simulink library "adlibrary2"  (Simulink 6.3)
undefined symbols (not defined in the file or in its folder): adlibrary2, ADM, DDRII, II, no_bitstream, SRAM, XP, XRC
libraries: xbsIndex_r4 x297, adlibrary2_d2sram_0 x5, adlibrary2 x5, adlibrary2_ddr_xpi0 x4, adlibrary2_ddr_xpl x3, adlibrary2_xpl32 x1, adlibrary2_xpl64 x1, adlibrary2_zbt64 x1, adlibrary2_zbt4_0 x1, adlibrary2_zbt4_1 x1, adlibrary2_zbt4_2 x1, adlibrary2_zbt4_3 x1
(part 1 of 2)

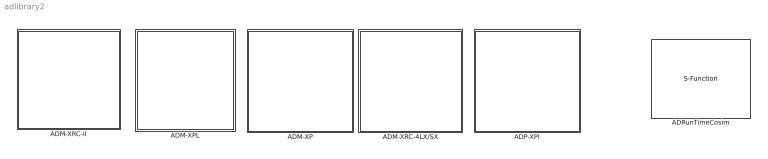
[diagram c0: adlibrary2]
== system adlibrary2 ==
  ADM-XP : Subsystem
  ADM-XPL : Subsystem
  ADM-XRC-4LX/SX : Subsystem  AncestorBlock=adlibrary2/ADM-XRC-II
  ADM-XRC-II : Subsystem
  ADP-XPI : Subsystem
  ADRunTimeCosim : S-Function  FunctionName=adcosim  Parameters='',index,bitstream,freq,single_step,shared  mask{index=0, bitstream=no_bitstream, freq=50, single_step=off, shared=None}
      mask prompts: index "Card Index"; freq "Clock Frequency"; single_step "Single Step"; shared "Share Access"

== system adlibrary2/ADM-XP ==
  DDR SDRAM 0 : Subsystem  mask{memsize=1}
      mask prompts: memsize "Simulation RAM Size (Mb)"
  DDR SDRAM 1 : Subsystem  mask{memsize=1}
      mask prompts: memsize "Simulation RAM Size (Mb)"
  DDRII SRAM 0 : Subsystem
  DDRII SRAM 1 : Subsystem  AncestorBlock=adlibrary2/ADM-XP/DDRII SRAM 0
  DDRII SRAM 2 : Subsystem
  DDRII SRAM 3 : Subsystem
  XPL 32 Bit Interface : adlibrary2/ADM-XPL/XPL 32 Bit Interface  program='load myprogram.txt'  clock_ratio=1.5
  XPL 64 Bit Interface : adlibrary2/ADM-XPL/XPL 64 Bit Interface  program='load myprogram.txt'  clock_ratio=1.5

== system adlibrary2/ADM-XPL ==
  DDR SDRAM : Subsystem  mask{memsize=1}
      mask prompts: memsize "Simulation RAM Size (Mb)"
  XPL 32 Bit Interface : Subsystem  mask{program='load myprogram.txt', clock_ratio=1.5}
      mask prompts: program "Local Bus Script Program"; clock_ratio "Clock Ratio"
  XPL 64 Bit Interface : Subsystem  mask{program='load myprogram.txt', clock_ratio=1.5}
      mask prompts: program "Local Bus Script Program"; clock_ratio "Clock Ratio"
  ZBT SRAM 64 : Subsystem

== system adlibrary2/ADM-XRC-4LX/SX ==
  PLX 32 Bit Interface : adlibrary2/ADM-XRC-II/PLX 32 Bit Interface  program='load myprogram.txt'  clock_ratio=1.5
  ZBT SRAM 0 : Subsystem
  ZBT SRAM 1 : Subsystem
  ZBT SRAM 2 : Subsystem
  ZBT SRAM 3 : Subsystem
  ZBT SRAM 4 : Subsystem
  ZBT SRAM 5 : Subsystem

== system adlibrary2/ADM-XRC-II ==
  PLX 32 Bit Interface : Subsystem  mask{program='load myprogram.txt', clock_ratio=1.5}
      mask prompts: program "Local Bus Script Program"; clock_ratio "Clock Ratio"
  "XRM DDR SDRAM " : Subsystem  mask{memsize=1}
      mask prompts: memsize "Simulation RAM Size (Mb)"
  ZBT SRAM 0 : Subsystem
  ZBT SRAM 1 : Subsystem
  ZBT SRAM 2 : Subsystem
  ZBT SRAM 3 : Subsystem
  ZBT SRAM 4 : Subsystem
  ZBT SRAM 5 : Subsystem

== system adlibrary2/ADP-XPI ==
  DDR SDRAM 0 : Subsystem  mask{memsize=1}
      mask prompts: memsize "Simulation RAM Size (Mb)"
  DDR SDRAM 1 : Subsystem  mask{memsize=1}
      mask prompts: memsize "Simulation RAM Size (Mb)"
  DDR SDRAM 2 : Subsystem  mask{memsize=1}
      mask prompts: memsize "Simulation RAM Size (Mb)"
  DDR SDRAM 3 : Subsystem  mask{memsize=1}
      mask prompts: memsize "Simulation RAM Size (Mb)"
  DDRII SRAM 0 : Subsystem
  XPL 32 Bit Interface : adlibrary2/ADM-XPL/XPL 32 Bit Interface  program='load myprogram.txt'  clock_ratio=1.5
  XPL 64 Bit Interface : adlibrary2/ADM-XPL/XPL 64 Bit Interface  program='load myprogram.txt'  clock_ratio=1.5

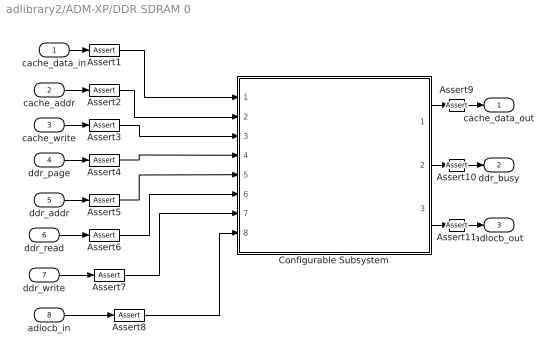
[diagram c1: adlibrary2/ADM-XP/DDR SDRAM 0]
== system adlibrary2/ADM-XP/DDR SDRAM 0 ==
  cache_data_in : Inport
  cache_addr : Inport  Port=2
  cache_write : Inport  Port=3
  ddr_page : Inport  Port=4
  ddr_addr : Inport  Port=5
  ddr_read : Inport  Port=6
  ddr_write : Inport  Port=7
  adlocb_in : Inport  Port=8
  Assert{1..11} (11 alike) : xbsIndex_r4/Assert  assert_type=off  type_source=Explicitly  arith_type="Signed  (2's comp)"  n_bits=16  bin_pt=14  assert_rate=on  rate_source=Explicitly  period=1  output_port=on  block_type=assert
  Configurable Subsystem : Subsystem  Tag=configX  BlockChoice=DDR SDRAM 32bit Simulation  mask{memsize=memsize}
      mask prompts: memsize "Simulation Ram Size (Mb)"
  cache_data_out : Outport
  ddr_busy : Outport  Port=2
  adlocb_out : Outport  Port=3
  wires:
  Configurable Subsystem/3(adlocb_out) -> Assert11/1
  Configurable Subsystem/2(ddr_busy) -> Assert10/1
  Configurable Subsystem/1(cache_data_out) -> Assert9/1
  cache_data_in/1 -> Assert1/1
  cache_addr/1 -> Assert2/1
  cache_write/1 -> Assert3/1
  ddr_page/1 -> Assert4/1
  ddr_addr/1 -> Assert5/1
  ddr_read/1 -> Assert6/1
  ddr_write/1 -> Assert7/1
  adlocb_in/1 -> Assert8/1
  Assert1/1 -> Configurable Subsystem/1(cache_data_in)
  Assert2/1 -> Configurable Subsystem/2(cache_addr)
  Assert3/1 -> Configurable Subsystem/3(cache_write)
  Assert4/1 -> Configurable Subsystem/4(ddr_page)
  Assert5/1 -> Configurable Subsystem/5(ddr_addr)
  Assert6/1 -> Configurable Subsystem/6(ddr_read)
  Assert7/1 -> Configurable Subsystem/7(ddr_write)
  Assert8/1 -> Configurable Subsystem/8(adlocb_in)
  Assert9/1 -> cache_data_out/1
  Assert10/1 -> ddr_busy/1
  Assert11/1 -> adlocb_out/1

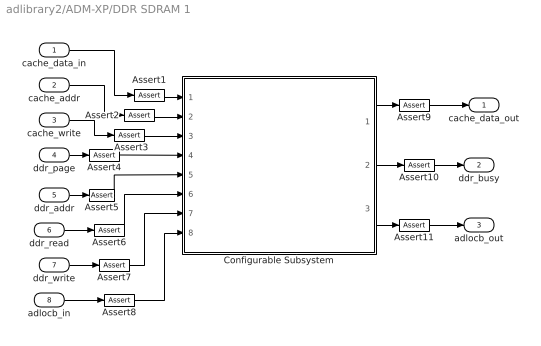
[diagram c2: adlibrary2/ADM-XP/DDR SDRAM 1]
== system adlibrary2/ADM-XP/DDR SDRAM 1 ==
  cache_data_in : Inport
  cache_addr : Inport  Port=2
  cache_write : Inport  Port=3
  ddr_page : Inport  Port=4
  ddr_addr : Inport  Port=5
  ddr_read : Inport  Port=6
  ddr_write : Inport  Port=7
  adlocb_in : Inport  Port=8
  Assert{1..11} (11 alike) : xbsIndex_r4/Assert  assert_type=off  type_source=Explicitly  arith_type="Signed  (2's comp)"  n_bits=16  bin_pt=14  assert_rate=on  rate_source=Explicitly  period=1  output_port=on  block_type=assert
  Configurable Subsystem : Subsystem  Tag=configX  BlockChoice=DDR SDRAM 32bit Simulation  mask{memsize=memsize}
      mask prompts: memsize "Simulation Ram Size (Mb)"
  cache_data_out : Outport
  ddr_busy : Outport  Port=2
  adlocb_out : Outport  Port=3
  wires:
  Configurable Subsystem/3(adlocb_out) -> Assert11/1
  Configurable Subsystem/2(ddr_busy) -> Assert10/1
  Configurable Subsystem/1(cache_data_out) -> Assert9/1
  cache_data_in/1 -> Assert1/1
  cache_addr/1 -> Assert2/1
  cache_write/1 -> Assert3/1
  ddr_page/1 -> Assert4/1
  ddr_addr/1 -> Assert5/1
  ddr_read/1 -> Assert6/1
  ddr_write/1 -> Assert7/1
  adlocb_in/1 -> Assert8/1
  Assert1/1 -> Configurable Subsystem/1(cache_data_in)
  Assert2/1 -> Configurable Subsystem/2(cache_addr)
  Assert3/1 -> Configurable Subsystem/3(cache_write)
  Assert4/1 -> Configurable Subsystem/4(ddr_page)
  Assert5/1 -> Configurable Subsystem/5(ddr_addr)
  Assert6/1 -> Configurable Subsystem/6(ddr_read)
  Assert7/1 -> Configurable Subsystem/7(ddr_write)
  Assert8/1 -> Configurable Subsystem/8(adlocb_in)
  Assert9/1 -> cache_data_out/1
  Assert10/1 -> ddr_busy/1
  Assert11/1 -> adlocb_out/1

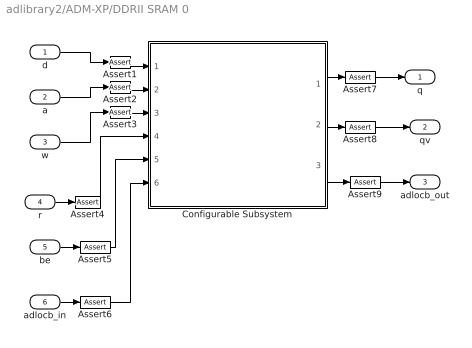
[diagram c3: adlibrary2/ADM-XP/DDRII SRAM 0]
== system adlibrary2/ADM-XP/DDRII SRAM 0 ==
  d : Inport
  a : Inport  Port=2
  w : Inport  Port=3
  r : Inport  Port=4
  be : Inport  Port=5
  adlocb_in : Inport  Port=6
  Assert{1..9} (9 alike) : xbsIndex_r4/Assert  assert_type=off  type_source=Explicitly  arith_type="Signed  (2's comp)"  n_bits=16  bin_pt=14  assert_rate=on  rate_source=Explicitly  period=1  output_port=on  block_type=assert
  Configurable Subsystem : Subsystem  Tag=configX  BlockChoice=DDRII SRAM Simulation
  q : Outport
  qv : Outport  Port=2
  adlocb_out : Outport  Port=3
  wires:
  Configurable Subsystem/1(q) -> Assert7/1
  d/1 -> Assert1/1
  a/1 -> Assert2/1
  w/1 -> Assert3/1
  r/1 -> Assert4/1
  be/1 -> Assert5/1
  adlocb_in/1 -> Assert6/1
  Configurable Subsystem/3(adlocb_out) -> Assert9/1
  Configurable Subsystem/2(qv) -> Assert8/1
  Assert1/1 -> Configurable Subsystem/1(d)
  Assert2/1 -> Configurable Subsystem/2(a)
  Assert3/1 -> Configurable Subsystem/3(w)
  Assert4/1 -> Configurable Subsystem/4(r)
  Assert5/1 -> Configurable Subsystem/5(be)
  Assert6/1 -> Configurable Subsystem/6(adlocb_in)
  Assert7/1 -> q/1
  Assert8/1 -> qv/1
  Assert9/1 -> adlocb_out/1

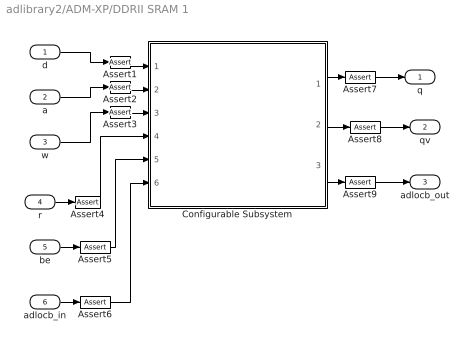
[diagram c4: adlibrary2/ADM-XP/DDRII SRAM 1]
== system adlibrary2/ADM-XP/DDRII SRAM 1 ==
  d : Inport
  a : Inport  Port=2
  w : Inport  Port=3
  r : Inport  Port=4
  be : Inport  Port=5
  adlocb_in : Inport  Port=6
  Assert{1..9} (9 alike) : xbsIndex_r4/Assert  assert_type=off  type_source=Explicitly  arith_type="Signed  (2's comp)"  n_bits=16  bin_pt=14  assert_rate=on  rate_source=Explicitly  period=1  output_port=on  block_type=assert
  Configurable Subsystem : Subsystem  Tag=configX  BlockChoice=DDRII SRAM Simulation
  q : Outport
  qv : Outport  Port=2
  adlocb_out : Outport  Port=3
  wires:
  Configurable Subsystem/1(q) -> Assert7/1
  d/1 -> Assert1/1
  a/1 -> Assert2/1
  w/1 -> Assert3/1
  r/1 -> Assert4/1
  be/1 -> Assert5/1
  adlocb_in/1 -> Assert6/1
  Configurable Subsystem/3(adlocb_out) -> Assert9/1
  Configurable Subsystem/2(qv) -> Assert8/1
  Assert1/1 -> Configurable Subsystem/1(d)
  Assert2/1 -> Configurable Subsystem/2(a)
  Assert3/1 -> Configurable Subsystem/3(w)
  Assert4/1 -> Configurable Subsystem/4(r)
  Assert5/1 -> Configurable Subsystem/5(be)
  Assert6/1 -> Configurable Subsystem/6(adlocb_in)
  Assert7/1 -> q/1
  Assert8/1 -> qv/1
  Assert9/1 -> adlocb_out/1

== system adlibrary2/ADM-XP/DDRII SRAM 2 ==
  d : Inport
  a : Inport  Port=2
  w : Inport  Port=3
  r : Inport  Port=4
  be : Inport  Port=5
  adlocb_in : Inport  Port=6
  Assert{1..9} (9 alike) : xbsIndex_r4/Assert  assert_type=off  type_source=Explicitly  arith_type="Signed  (2's comp)"  n_bits=16  bin_pt=14  assert_rate=on  rate_source=Explicitly  period=1  output_port=on  block_type=assert
  Configurable Subsystem : Subsystem  Tag=configX  BlockChoice=DDRII SRAM Simulation
  q : Outport
  qv : Outport  Port=2
  adlocb_out : Outport  Port=3
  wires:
  Configurable Subsystem/2(qv) -> Assert2/1
  Configurable Subsystem/3(adlocb_out) -> Assert3/1
  adlocb_in/1 -> Assert9/1
  be/1 -> Assert8/1
  r/1 -> Assert7/1
  w/1 -> Assert6/1
  a/1 -> Assert5/1
  d/1 -> Assert4/1
  Configurable Subsystem/1(q) -> Assert1/1
  Assert1/1 -> q/1
  Assert2/1 -> qv/1
  Assert3/1 -> adlocb_out/1
  Assert4/1 -> Configurable Subsystem/1(d)
  Assert5/1 -> Configurable Subsystem/2(a)
  Assert6/1 -> Configurable Subsystem/3(w)
  Assert7/1 -> Configurable Subsystem/4(r)
  Assert8/1 -> Configurable Subsystem/5(be)
  Assert9/1 -> Configurable Subsystem/6(adlocb_in)

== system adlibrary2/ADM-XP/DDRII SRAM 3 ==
  d : Inport
  a : Inport  Port=2
  w : Inport  Port=3
  r : Inport  Port=4
  be : Inport  Port=5
  adlocb_in : Inport  Port=6
  Assert{1..9} (9 alike) : xbsIndex_r4/Assert  assert_type=off  type_source=Explicitly  arith_type="Signed  (2's comp)"  n_bits=16  bin_pt=14  assert_rate=on  rate_source=Explicitly  period=1  output_port=on  block_type=assert
  Configurable Subsystem : Subsystem  Tag=configX  BlockChoice=DDRII SRAM Simulation
  q : Outport
  qv : Outport  Port=2
  adlocb_out : Outport  Port=3
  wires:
  Configurable Subsystem/2(qv) -> Assert8/1
  Configurable Subsystem/3(adlocb_out) -> Assert9/1
  adlocb_in/1 -> Assert6/1
  be/1 -> Assert5/1
  r/1 -> Assert4/1
  w/1 -> Assert3/1
  a/1 -> Assert2/1
  d/1 -> Assert1/1
  Configurable Subsystem/1(q) -> Assert7/1
  Assert1/1 -> Configurable Subsystem/1(d)
  Assert2/1 -> Configurable Subsystem/2(a)
  Assert3/1 -> Configurable Subsystem/3(w)
  Assert4/1 -> Configurable Subsystem/4(r)
  Assert5/1 -> Configurable Subsystem/5(be)
  Assert6/1 -> Configurable Subsystem/6(adlocb_in)
  Assert7/1 -> q/1
  Assert8/1 -> qv/1
  Assert9/1 -> adlocb_out/1

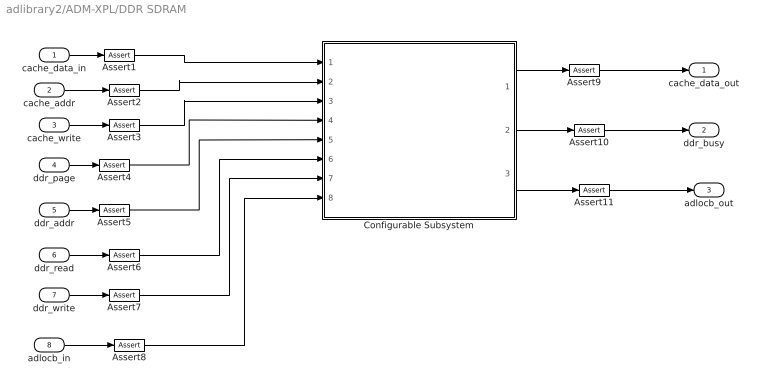
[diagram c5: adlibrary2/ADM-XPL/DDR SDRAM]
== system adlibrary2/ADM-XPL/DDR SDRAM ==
  cache_data_in : Inport
  cache_addr : Inport  Port=2
  cache_write : Inport  Port=3
  ddr_page : Inport  Port=4
  ddr_addr : Inport  Port=5
  ddr_read : Inport  Port=6
  ddr_write : Inport  Port=7
  adlocb_in : Inport  Port=8
  Assert{1..11} (11 alike) : xbsIndex_r4/Assert  assert_type=off  type_source=Explicitly  arith_type="Signed  (2's comp)"  n_bits=16  bin_pt=14  assert_rate=on  rate_source=Explicitly  period=1  output_port=on  block_type=assert
  Configurable Subsystem : Subsystem  Tag=configX  BlockChoice=DDR SDRAM 32bit Simulation  mask{memsize=memsize}
      mask prompts: memsize "Simulation Ram Size (Mb)"
  cache_data_out : Outport
  ddr_busy : Outport  Port=2
  adlocb_out : Outport  Port=3
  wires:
  cache_data_in/1 -> Assert1/1
  cache_addr/1 -> Assert2/1
  cache_write/1 -> Assert3/1
  ddr_page/1 -> Assert4/1
  ddr_addr/1 -> Assert5/1
  ddr_read/1 -> Assert6/1
  ddr_write/1 -> Assert7/1
  adlocb_in/1 -> Assert8/1
  Configurable Subsystem/1(cache_data_out) -> Assert9/1
  Configurable Subsystem/2(ddr_busy) -> Assert10/1
  Configurable Subsystem/3(adlocb_out) -> Assert11/1
  Assert1/1 -> Configurable Subsystem/1(cache_data_in)
  Assert2/1 -> Configurable Subsystem/2(cache_addr)
  Assert3/1 -> Configurable Subsystem/3(cache_write)
  Assert4/1 -> Configurable Subsystem/4(ddr_page)
  Assert5/1 -> Configurable Subsystem/5(ddr_addr)
  Assert6/1 -> Configurable Subsystem/6(ddr_read)
  Assert7/1 -> Configurable Subsystem/7(ddr_write)
  Assert8/1 -> Configurable Subsystem/8(adlocb_in)
  Assert9/1 -> cache_data_out/1
  Assert10/1 -> ddr_busy/1
  Assert11/1 -> adlocb_out/1

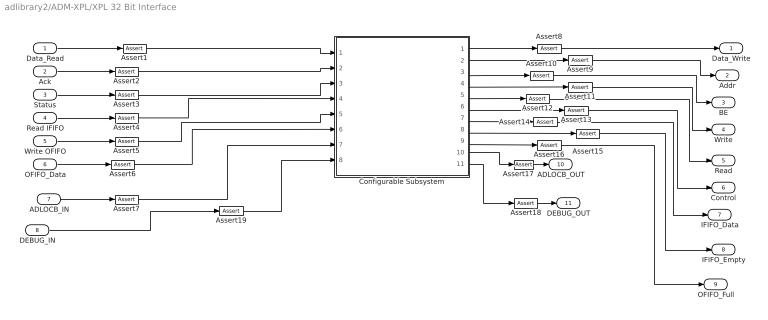
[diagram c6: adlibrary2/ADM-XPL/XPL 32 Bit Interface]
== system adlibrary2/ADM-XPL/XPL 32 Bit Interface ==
  Data_Read : Inport
  Ack : Inport  Port=2
  Status : Inport  Port=3
  Read IFIFO : Inport  Port=4
  Write OFIFO : Inport  Port=5
  OFIFO_Data : Inport  Port=6
  ADLOCB_IN : Inport  Port=7
  DEBUG_IN : Inport  Port=8
  Assert{1..19} (19 alike) : xbsIndex_r4/Assert  assert_type=off  type_source=Explicitly  arith_type="Signed  (2's comp)"  n_bits=16  bin_pt=14  assert_rate=on  rate_source=Explicitly  period=1  output_port=on  block_type=assert
  Configurable Subsystem : Subsystem  Tag=configX  BlockChoice=XPL 32Bit Simulation  mask{program=program, clock_ratio=clock_ratio}
      mask prompts: program "Local Bus Script Program"; clock_ratio "Clock Ratio"
  Data_Write : Outport
  Addr : Outport  Port=2
  BE : Outport  Port=3
  Write : Outport  Port=4
  Read : Outport  Port=5
  Control : Outport  Port=6
  IFIFO_Data : Outport  Port=7
  IFIFO_Empty : Outport  Port=8
  OFIFO_Full : Outport  Port=9
  ADLOCB_OUT : Outport  Port=10
  DEBUG_OUT : Outport  Port=11
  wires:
  Status/1 -> Assert3/1
  Ack/1 -> Assert2/1
  Data_Read/1 -> Assert1/1
  Configurable Subsystem/9(OFIFO_Full) -> Assert16/1
  Configurable Subsystem/8(IFIFO_Empty) -> Assert15/1
  Configurable Subsystem/7(IFIFO_Data) -> Assert14/1
  Configurable Subsystem/6(Control) -> Assert13/1
  Configurable Subsystem/5(Read) -> Assert12/1
  Configurable Subsystem/4(Write) -> Assert11/1
  Configurable Subsystem/3(BE) -> Assert10/1
  Configurable Subsystem/1(Data_Write) -> Assert8/1
  Configurable Subsystem/2(Addr) -> Assert9/1
  Read IFIFO/1 -> Assert4/1
  Write OFIFO/1 -> Assert5/1
  OFIFO_Data/1 -> Assert6/1
  ADLOCB_IN/1 -> Assert7/1
  Configurable Subsystem/10(ADLOCB_OUT) -> Assert17/1
  Assert1/1 -> Configurable Subsystem/1(Data_Read)
  Assert2/1 -> Configurable Subsystem/2(Ack)
  Assert3/1 -> Configurable Subsystem/3(Status)
  Assert4/1 -> Configurable Subsystem/4(Read IFIFO)
  Assert8/1 -> Data_Write/1
  Assert9/1 -> Addr/1
  Assert10/1 -> BE/1
  Assert11/1 -> Write/1
  Assert12/1 -> Read/1
  Assert13/1 -> Control/1
  Assert14/1 -> IFIFO_Data/1
  Assert15/1 -> IFIFO_Empty/1
  Assert16/1 -> OFIFO_Full/1
  Assert17/1 -> ADLOCB_OUT/1
  Assert5/1 -> Configurable Subsystem/5(Write OFIFO)
  Assert6/1 -> Configurable Subsystem/6(OFIFO_Data)
  Assert7/1 -> Configurable Subsystem/7(ADLOCB_IN)
  DEBUG_IN/1 -> Assert19/1
  Assert19/1 -> Configurable Subsystem/8(DEBUG_IN)
  Assert18/1 -> DEBUG_OUT/1
  Configurable Subsystem/11(DEBUG_OUT) -> Assert18/1

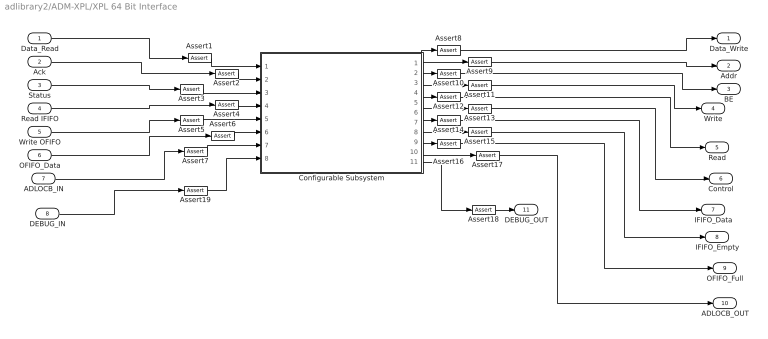
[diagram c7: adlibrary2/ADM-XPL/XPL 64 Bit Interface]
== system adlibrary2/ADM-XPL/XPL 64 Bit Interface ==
  Data_Read : Inport
  Ack : Inport  Port=2
  Status : Inport  Port=3
  Read IFIFO : Inport  Port=4
  Write OFIFO : Inport  Port=5
  OFIFO_Data : Inport  Port=6
  ADLOCB_IN : Inport  Port=7
  DEBUG_IN : Inport  Port=8
  Assert{1..19} (19 alike) : xbsIndex_r4/Assert  assert_type=off  type_source=Explicitly  arith_type="Signed  (2's comp)"  n_bits=16  bin_pt=14  assert_rate=on  rate_source=Explicitly  period=1  output_port=on  block_type=assert
  Configurable Subsystem : Subsystem  Tag=configX  BlockChoice=XPL 64Bit Simulation  mask{program=program, clock_ratio=clock_ratio}
      mask prompts: program "Local Bus Script Program"; clock_ratio "Clock Ratio"
  Data_Write : Outport
  Addr : Outport  Port=2
  BE : Outport  Port=3
  Write : Outport  Port=4
  Read : Outport  Port=5
  Control : Outport  Port=6
  IFIFO_Data : Outport  Port=7
  IFIFO_Empty : Outport  Port=8
  OFIFO_Full : Outport  Port=9
  ADLOCB_OUT : Outport  Port=10
  DEBUG_OUT : Outport  Port=11
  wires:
  Configurable Subsystem/1(Data_Write) -> Assert8/1
  Configurable Subsystem/2(Addr) -> Assert9/1
  Configurable Subsystem/4(Write) -> Assert11/1
  Configurable Subsystem/5(Read) -> Assert12/1
  Configurable Subsystem/6(Control) -> Assert13/1
  Configurable Subsystem/7(IFIFO_Data) -> Assert14/1
  Configurable Subsystem/8(IFIFO_Empty) -> Assert15/1
  Configurable Subsystem/9(OFIFO_Full) -> Assert16/1
  Data_Read/1 -> Assert1/1
  Ack/1 -> Assert2/1
  Status/1 -> Assert3/1
  Read IFIFO/1 -> Assert4/1
  Write OFIFO/1 -> Assert5/1
  OFIFO_Data/1 -> Assert6/1
  ADLOCB_IN/1 -> Assert7/1
  Configurable Subsystem/3(BE) -> Assert10/1
  Configurable Subsystem/10(ADLOCB_OUT) -> Assert17/1
  Assert1/1 -> Configurable Subsystem/1(Data_Read)
  Assert2/1 -> Configurable Subsystem/2(Ack)
  Assert3/1 -> Configurable Subsystem/3(Status)
  Assert4/1 -> Configurable Subsystem/4(Read IFIFO)
  Assert5/1 -> Configurable Subsystem/5(Write OFIFO)
  Assert6/1 -> Configurable Subsystem/6(OFIFO_Data)
  Assert7/1 -> Configurable Subsystem/7(ADLOCB_IN)
  Assert8/1 -> Data_Write/1
  Assert9/1 -> Addr/1
  Assert10/1 -> BE/1
  Assert11/1 -> Write/1
  Assert12/1 -> Read/1
  Assert13/1 -> Control/1
  Assert14/1 -> IFIFO_Data/1
  Assert15/1 -> IFIFO_Empty/1
  Assert16/1 -> OFIFO_Full/1
  Assert17/1 -> ADLOCB_OUT/1
  Assert18/1 -> DEBUG_OUT/1
  Configurable Subsystem/11(DEBUG_OUT) -> Assert18/1
  Assert19/1 -> Configurable Subsystem/8(DEBUG_IN)
  DEBUG_IN/1 -> Assert19/1

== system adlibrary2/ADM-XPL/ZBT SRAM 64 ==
  d : Inport
  a : Inport  Port=2
  w : Inport  Port=3
  r : Inport  Port=4
  be : Inport  Port=5
  adlocb_in : Inport  Port=6
  Assert{1..9} (9 alike) : xbsIndex_r4/Assert  assert_type=off  type_source=Explicitly  arith_type="Signed  (2's comp)"  n_bits=16  bin_pt=14  assert_rate=on  rate_source=Explicitly  period=1  output_port=on  block_type=assert
  Configurable Subsystem : Subsystem  Tag=configX  BlockChoice=ZBT SRAM 64bit Simulation
  q : Outport
  qv : Outport  Port=2
  adlocb_out : Outport  Port=3
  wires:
  d/1 -> Assert1/1
  a/1 -> Assert2/1
  w/1 -> Assert3/1
  r/1 -> Assert4/1
  be/1 -> Assert5/1
  adlocb_in/1 -> Assert6/1
  Configurable Subsystem/1(q) -> Assert7/1
  Configurable Subsystem/2(qv) -> Assert8/1
  Configurable Subsystem/3(adlocb_out) -> Assert9/1
  Assert1/1 -> Configurable Subsystem/1(d)
  Assert2/1 -> Configurable Subsystem/2(a)
  Assert3/1 -> Configurable Subsystem/3(w)
  Assert4/1 -> Configurable Subsystem/4(r)
  Assert5/1 -> Configurable Subsystem/5(be)
  Assert6/1 -> Configurable Subsystem/6(adlocb_in)
  Assert7/1 -> q/1
  Assert8/1 -> qv/1
  Assert9/1 -> adlocb_out/1

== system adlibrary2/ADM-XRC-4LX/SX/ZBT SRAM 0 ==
  d : Inport
  a : Inport  Port=2
  w : Inport  Port=3
  r : Inport  Port=4
  be : Inport  Port=5
  adlocb_in : Inport  Port=6
  Assert{1..9} (9 alike) : xbsIndex_r4/Assert  assert_type=off  type_source=Explicitly  arith_type="Signed  (2's comp)"  n_bits=16  bin_pt=14  assert_rate=on  rate_source=Explicitly  period=1  output_port=on  block_type=assert
  Configurable Subsystem : Subsystem  Tag=configX  BlockChoice=ZBT SRAM 32Bit Simulation
  q : Outport
  qv : Outport  Port=2
  adlocb_out : Outport  Port=3
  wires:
  Configurable Subsystem/3(adlocb_out) -> Assert9/1
  Configurable Subsystem/2(qv) -> Assert8/1
  Configurable Subsystem/1(q) -> Assert7/1
  adlocb_in/1 -> Assert6/1
  be/1 -> Assert5/1
  r/1 -> Assert4/1
  w/1 -> Assert3/1
  a/1 -> Assert2/1
  d/1 -> Assert1/1
  Assert1/1 -> Configurable Subsystem/1(d)
  Assert2/1 -> Configurable Subsystem/2(a)
  Assert3/1 -> Configurable Subsystem/3(w)
  Assert4/1 -> Configurable Subsystem/4(r)
  Assert5/1 -> Configurable Subsystem/5(be)
  Assert6/1 -> Configurable Subsystem/6(adlocb_in)
  Assert7/1 -> q/1
  Assert8/1 -> qv/1
  Assert9/1 -> adlocb_out/1

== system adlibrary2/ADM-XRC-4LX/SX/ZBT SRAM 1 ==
  d : Inport
  a : Inport  Port=2
  w : Inport  Port=3
  r : Inport  Port=4
  be : Inport  Port=5
  adlocb_in : Inport  Port=6
  Assert{1..9} (9 alike) : xbsIndex_r4/Assert  assert_type=off  type_source=Explicitly  arith_type="Signed  (2's comp)"  n_bits=16  bin_pt=14  assert_rate=on  rate_source=Explicitly  period=1  output_port=on  block_type=assert
  Configurable Subsystem : Subsystem  Tag=configX  BlockChoice=ZBT SRAM 32Bit Simulation
  q : Outport
  qv : Outport  Port=2
  adlocb_out : Outport  Port=3
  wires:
  d/1 -> Assert1/1
  a/1 -> Assert2/1
  w/1 -> Assert3/1
  r/1 -> Assert4/1
  be/1 -> Assert5/1
  adlocb_in/1 -> Assert6/1
  Configurable Subsystem/1(q) -> Assert7/1
  Configurable Subsystem/2(qv) -> Assert8/1
  Configurable Subsystem/3(adlocb_out) -> Assert9/1
  Assert1/1 -> Configurable Subsystem/1(d)
  Assert2/1 -> Configurable Subsystem/2(a)
  Assert3/1 -> Configurable Subsystem/3(w)
  Assert4/1 -> Configurable Subsystem/4(r)
  Assert5/1 -> Configurable Subsystem/5(be)
  Assert6/1 -> Configurable Subsystem/6(adlocb_in)
  Assert7/1 -> q/1
  Assert8/1 -> qv/1
  Assert9/1 -> adlocb_out/1

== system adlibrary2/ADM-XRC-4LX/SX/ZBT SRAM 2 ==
  d : Inport
  a : Inport  Port=2
  w : Inport  Port=3
  r : Inport  Port=4
  be : Inport  Port=5
  adlocb_in : Inport  Port=6
  Assert{1..9} (9 alike) : xbsIndex_r4/Assert  assert_type=off  type_source=Explicitly  arith_type="Signed  (2's comp)"  n_bits=16  bin_pt=14  assert_rate=on  rate_source=Explicitly  period=1  output_port=on  block_type=assert
  Configurable Subsystem : Subsystem  Tag=configX  BlockChoice=ZBT SRAM 32Bit Simulation
  q : Outport
  qv : Outport  Port=2
  adlocb_out : Outport  Port=3
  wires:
  d/1 -> Assert1/1
  a/1 -> Assert2/1
  w/1 -> Assert3/1
  r/1 -> Assert4/1
  be/1 -> Assert5/1
  adlocb_in/1 -> Assert6/1
  Configurable Subsystem/1(q) -> Assert8/1
  Configurable Subsystem/2(qv) -> Assert9/1
  Configurable Subsystem/3(adlocb_out) -> Assert7/1
  Assert1/1 -> Configurable Subsystem/1(d)
  Assert2/1 -> Configurable Subsystem/2(a)
  Assert3/1 -> Configurable Subsystem/3(w)
  Assert4/1 -> Configurable Subsystem/4(r)
  Assert5/1 -> Configurable Subsystem/5(be)
  Assert6/1 -> Configurable Subsystem/6(adlocb_in)
  Assert7/1 -> adlocb_out/1
  Assert8/1 -> q/1
  Assert9/1 -> qv/1

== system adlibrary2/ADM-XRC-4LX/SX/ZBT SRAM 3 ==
  d : Inport
  a : Inport  Port=2
  w : Inport  Port=3
  r : Inport  Port=4
  be : Inport  Port=5
  adlocb_in : Inport  Port=6
  Assert{1..9} (9 alike) : xbsIndex_r4/Assert  assert_type=off  type_source=Explicitly  arith_type="Signed  (2's comp)"  n_bits=16  bin_pt=14  assert_rate=on  rate_source=Explicitly  period=1  output_port=on  block_type=assert
  Configurable Subsystem : Subsystem  Tag=configX  BlockChoice=ZBT SRAM 32Bit Simulation
  q : Outport
  qv : Outport  Port=2
  adlocb_out : Outport  Port=3
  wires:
  d/1 -> Assert1/1
  a/1 -> Assert2/1
  w/1 -> Assert3/1
  r/1 -> Assert4/1
  be/1 -> Assert5/1
  adlocb_in/1 -> Assert6/1
  Configurable Subsystem/1(q) -> Assert7/1
  Configurable Subsystem/2(qv) -> Assert8/1
  Configurable Subsystem/3(adlocb_out) -> Assert9/1
  Assert1/1 -> Configurable Subsystem/1(d)
  Assert2/1 -> Configurable Subsystem/2(a)
  Assert3/1 -> Configurable Subsystem/3(w)
  Assert4/1 -> Configurable Subsystem/4(r)
  Assert5/1 -> Configurable Subsystem/5(be)
  Assert6/1 -> Configurable Subsystem/6(adlocb_in)
  Assert7/1 -> q/1
  Assert8/1 -> qv/1
  Assert9/1 -> adlocb_out/1

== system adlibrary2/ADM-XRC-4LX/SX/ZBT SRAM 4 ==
  d : Inport
  a : Inport  Port=2
  w : Inport  Port=3
  r : Inport  Port=4
  be : Inport  Port=5
  adlocb_in : Inport  Port=6
  Assert{1..9} (9 alike) : xbsIndex_r4/Assert  assert_type=off  type_source=Explicitly  arith_type="Signed  (2's comp)"  n_bits=16  bin_pt=14  assert_rate=on  rate_source=Explicitly  period=1  output_port=on  block_type=assert
  Configurable Subsystem : Subsystem  Tag=configX  BlockChoice=ZBT SRAM 32Bit Simulation
  q : Outport
  qv : Outport  Port=2
  adlocb_out : Outport  Port=3
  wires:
  d/1 -> Assert1/1
  a/1 -> Assert2/1
  w/1 -> Assert3/1
  r/1 -> Assert4/1
  be/1 -> Assert5/1
  adlocb_in/1 -> Assert6/1
  Configurable Subsystem/1(q) -> Assert7/1
  Configurable Subsystem/2(qv) -> Assert8/1
  Configurable Subsystem/3(adlocb_out) -> Assert9/1
  Assert1/1 -> Configurable Subsystem/1(d)
  Assert2/1 -> Configurable Subsystem/2(a)
  Assert3/1 -> Configurable Subsystem/3(w)
  Assert4/1 -> Configurable Subsystem/4(r)
  Assert5/1 -> Configurable Subsystem/5(be)
  Assert6/1 -> Configurable Subsystem/6(adlocb_in)
  Assert7/1 -> q/1
  Assert8/1 -> qv/1
  Assert9/1 -> adlocb_out/1

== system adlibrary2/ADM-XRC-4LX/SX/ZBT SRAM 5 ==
  d : Inport
  a : Inport  Port=2
  w : Inport  Port=3
  r : Inport  Port=4
  be : Inport  Port=5
  adlocb_in : Inport  Port=6
  Assert{1..9} (9 alike) : xbsIndex_r4/Assert  assert_type=off  type_source=Explicitly  arith_type="Signed  (2's comp)"  n_bits=16  bin_pt=14  assert_rate=on  rate_source=Explicitly  period=1  output_port=on  block_type=assert
  Configurable Subsystem : Subsystem  Tag=configX  BlockChoice=ZBT SRAM 32Bit Simulation
  q : Outport
  qv : Outport  Port=2
  adlocb_out : Outport  Port=3
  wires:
  d/1 -> Assert1/1
  a/1 -> Assert2/1
  w/1 -> Assert3/1
  r/1 -> Assert4/1
  be/1 -> Assert5/1
  adlocb_in/1 -> Assert6/1
  Configurable Subsystem/1(q) -> Assert7/1
  Configurable Subsystem/2(qv) -> Assert8/1
  Configurable Subsystem/3(adlocb_out) -> Assert9/1
  Assert1/1 -> Configurable Subsystem/1(d)
  Assert2/1 -> Configurable Subsystem/2(a)
  Assert3/1 -> Configurable Subsystem/3(w)
  Assert4/1 -> Configurable Subsystem/4(r)
  Assert5/1 -> Configurable Subsystem/5(be)
  Assert6/1 -> Configurable Subsystem/6(adlocb_in)
  Assert7/1 -> q/1
  Assert8/1 -> qv/1
  Assert9/1 -> adlocb_out/1

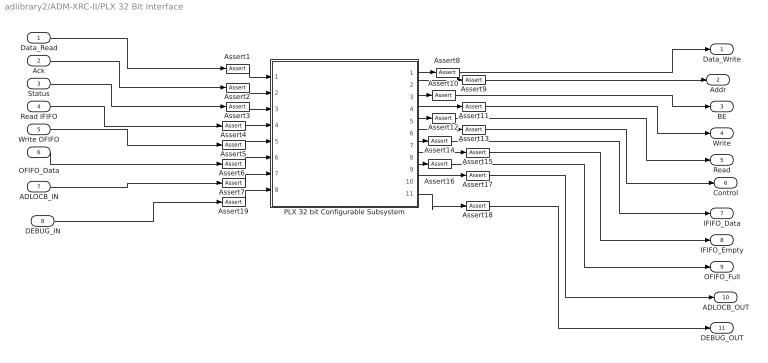
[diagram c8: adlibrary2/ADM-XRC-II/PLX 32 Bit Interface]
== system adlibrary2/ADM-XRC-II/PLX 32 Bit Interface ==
  Data_Read : Inport
  Ack : Inport  Port=2
  Status : Inport  Port=3
  Read IFIFO : Inport  Port=4
  Write OFIFO : Inport  Port=5
  OFIFO_Data : Inport  Port=6
  ADLOCB_IN : Inport  Port=7
  DEBUG_IN : Inport  Port=8
  Assert{1..19} (19 alike) : xbsIndex_r4/Assert  assert_type=off  type_source=Explicitly  arith_type="Signed  (2's comp)"  n_bits=16  bin_pt=14  assert_rate=on  rate_source=Explicitly  period=1  output_port=on  block_type=assert
  PLX 32 bit Configurable Subsystem : Subsystem  Tag=configX  BlockChoice=PLX 32Bit Simulation  mask{program=program, clock_ratio=clock_ratio}
      mask prompts: program "Local Bus Script Program"; clock_ratio "Clock Ratio"
  Data_Write : Outport
  Addr : Outport  Port=2
  BE : Outport  Port=3
  Write : Outport  Port=4
  Read : Outport  Port=5
  Control : Outport  Port=6
  IFIFO_Data : Outport  Port=7
  IFIFO_Empty : Outport  Port=8
  OFIFO_Full : Outport  Port=9
  ADLOCB_OUT : Outport  Port=10
  DEBUG_OUT : Outport  Port=11
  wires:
  PLX 32 bit Configurable Subsystem/1(Data_Write) -> Assert8/1
  PLX 32 bit Configurable Subsystem/2(Addr) -> Assert9/1
  PLX 32 bit Configurable Subsystem/4(Write) -> Assert11/1
  PLX 32 bit Configurable Subsystem/6(Control) -> Assert13/1
  PLX 32 bit Configurable Subsystem/7(IFIFO_Data) -> Assert14/1
  PLX 32 bit Configurable Subsystem/8(IFIFO_Empty) -> Assert15/1
  PLX 32 bit Configurable Subsystem/9(OFIFO_Full) -> Assert16/1
  PLX 32 bit Configurable Subsystem/3(BE) -> Assert10/1
  PLX 32 bit Configurable Subsystem/10(ADLOCB_OUT) -> Assert17/1
  Data_Read/1 -> Assert1/1
  Ack/1 -> Assert2/1
  Status/1 -> Assert3/1
  Read IFIFO/1 -> Assert4/1
  Write OFIFO/1 -> Assert5/1
  OFIFO_Data/1 -> Assert6/1
  ADLOCB_IN/1 -> Assert7/1
  PLX 32 bit Configurable Subsystem/5(Read) -> Assert12/1
  Assert1/1 -> PLX 32 bit Configurable Subsystem/1(Data_Read)
  Assert2/1 -> PLX 32 bit Configurable Subsystem/2(Ack)
  Assert3/1 -> PLX 32 bit Configurable Subsystem/3(Status)
  Assert4/1 -> PLX 32 bit Configurable Subsystem/4(Read IFIFO)
  Assert5/1 -> PLX 32 bit Configurable Subsystem/5(Write OFIFO)
  Assert6/1 -> PLX 32 bit Configurable Subsystem/6(OFIFO_Data)
  Assert7/1 -> PLX 32 bit Configurable Subsystem/7(ADLOCB_IN)
  Assert8/1 -> Data_Write/1
  Assert9/1 -> Addr/1
  Assert10/1 -> BE/1
  Assert11/1 -> Write/1
  Assert12/1 -> Read/1
  Assert13/1 -> Control/1
  Assert14/1 -> IFIFO_Data/1
  Assert15/1 -> IFIFO_Empty/1
  Assert16/1 -> OFIFO_Full/1
  Assert17/1 -> ADLOCB_OUT/1
  DEBUG_IN/1 -> Assert19/1
  PLX 32 bit Configurable Subsystem/11(DEBUG_OUT) -> Assert18/1
  Assert18/1 -> DEBUG_OUT/1
  Assert19/1 -> PLX 32 bit Configurable Subsystem/8(DEBUG_IN)

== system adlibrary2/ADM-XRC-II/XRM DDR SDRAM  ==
  cache_data_in : Inport
  cache_addr : Inport  Port=2
  cache_write : Inport  Port=3
  ddr_page : Inport  Port=4
  ddr_addr : Inport  Port=5
  ddr_read : Inport  Port=6
  ddr_write : Inport  Port=7
  Assert{1..9} (9 alike) : xbsIndex_r4/Assert  assert_type=off  type_source=Explicitly  arith_type="Signed  (2's comp)"  n_bits=16  bin_pt=14  assert_rate=on  rate_source=Explicitly  period=1  output_port=on  block_type=assert
  Configurable Subsystem : Subsystem  Tag=configX  BlockChoice=DDR SDRAM 64bit Simulation
  cache_data_out : Outport
  ddr_busy : Outport  Port=2
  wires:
  cache_data_in/1 -> Assert1/1
  cache_addr/1 -> Assert2/1
  cache_write/1 -> Assert3/1
  ddr_page/1 -> Assert4/1
  ddr_addr/1 -> Assert5/1
  ddr_read/1 -> Assert6/1
  ddr_write/1 -> Assert7/1
  Configurable Subsystem/1(cache_data_out) -> Assert8/1
  Configurable Subsystem/2(ddr_busy) -> Assert9/1
  Assert1/1 -> Configurable Subsystem/1(cache_data_in)
  Assert2/1 -> Configurable Subsystem/2(cache_addr)
  Assert3/1 -> Configurable Subsystem/3(cache_write)
  Assert4/1 -> Configurable Subsystem/4(ddr_page)
  Assert5/1 -> Configurable Subsystem/5(ddr_addr)
  Assert6/1 -> Configurable Subsystem/6(ddr_read)
  Assert7/1 -> Configurable Subsystem/7(ddr_write)
  Assert8/1 -> cache_data_out/1
  Assert9/1 -> ddr_busy/1

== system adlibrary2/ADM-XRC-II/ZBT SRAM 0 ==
  d : Inport
  a : Inport  Port=2
  w : Inport  Port=3
  r : Inport  Port=4
  be : Inport  Port=5
  adlocb_in : Inport  Port=6
  Assert{,1..8} (9 alike) : xbsIndex_r4/Assert  assert_type=off  type_source=Explicitly  arith_type="Signed  (2's comp)"  n_bits=16  bin_pt=14  assert_rate=on  rate_source=Explicitly  period=1  output_port=on  block_type=assert
  Configurable Subsystem : Subsystem  Tag=configX  BlockChoice=ZBT SRAM 32Bit Simulation
  q : Outport
  qv : Outport  Port=2
  adlocb_out : Outport  Port=3
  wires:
  d/1 -> Assert/1
  a/1 -> Assert1/1
  w/1 -> Assert2/1
  r/1 -> Assert3/1
  be/1 -> Assert4/1
  adlocb_in/1 -> Assert5/1
  Configurable Subsystem/1(q) -> Assert8/1
  Configurable Subsystem/2(qv) -> Assert7/1
  Configurable Subsystem/3(adlocb_out) -> Assert6/1
  Assert/1 -> Configurable Subsystem/1(d)
  Assert1/1 -> Configurable Subsystem/2(a)
  Assert2/1 -> Configurable Subsystem/3(w)
  Assert3/1 -> Configurable Subsystem/4(r)
  Assert4/1 -> Configurable Subsystem/5(be)
  Assert5/1 -> Configurable Subsystem/6(adlocb_in)
  Assert6/1 -> adlocb_out/1
  Assert7/1 -> qv/1
  Assert8/1 -> q/1

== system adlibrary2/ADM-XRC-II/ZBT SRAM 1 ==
  d : Inport
  a : Inport  Port=2
  w : Inport  Port=3
  r : Inport  Port=4
  be : Inport  Port=5
  adlocb_in : Inport  Port=6
  Assert{,2..9} (9 alike) : xbsIndex_r4/Assert  assert_type=off  type_source=Explicitly  arith_type="Signed  (2's comp)"  n_bits=16  bin_pt=14  assert_rate=on  rate_source=Explicitly  period=1  output_port=on  block_type=assert
  Configurable Subsystem : Subsystem  Tag=configX  BlockChoice=ZBT SRAM 32Bit Simulation
  q : Outport
  qv : Outport  Port=2
  adlocb_out : Outport  Port=3
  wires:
  Configurable Subsystem/3(adlocb_out) -> Assert9/1
  Configurable Subsystem/2(qv) -> Assert8/1
  Configurable Subsystem/1(q) -> Assert7/1
  adlocb_in/1 -> Assert6/1
  be/1 -> Assert5/1
  r/1 -> Assert4/1
  w/1 -> Assert3/1
  a/1 -> Assert2/1
  d/1 -> Assert/1
  Assert/1 -> Configurable Subsystem/1(d)
  Assert2/1 -> Configurable Subsystem/2(a)
  Assert3/1 -> Configurable Subsystem/3(w)
  Assert4/1 -> Configurable Subsystem/4(r)
  Assert5/1 -> Configurable Subsystem/5(be)
  Assert6/1 -> Configurable Subsystem/6(adlocb_in)
  Assert7/1 -> q/1
  Assert8/1 -> qv/1
  Assert9/1 -> adlocb_out/1

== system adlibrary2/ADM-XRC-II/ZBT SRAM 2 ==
  d : Inport
  a : Inport  Port=2
  w : Inport  Port=3
  r : Inport  Port=4
  be : Inport  Port=5
  adlocb_in : Inport  Port=6
  Assert{1..9} (9 alike) : xbsIndex_r4/Assert  assert_type=off  type_source=Explicitly  arith_type="Signed  (2's comp)"  n_bits=16  bin_pt=14  assert_rate=on  rate_source=Explicitly  period=1  output_port=on  block_type=assert
  Configurable Subsystem : Subsystem  Tag=configX  BlockChoice=ZBT SRAM 32Bit Simulation
  q : Outport
  qv : Outport  Port=2
  adlocb_out : Outport  Port=3
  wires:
  Configurable Subsystem/3(adlocb_out) -> Assert9/1
  Configurable Subsystem/2(qv) -> Assert8/1
  Configurable Subsystem/1(q) -> Assert7/1
  adlocb_in/1 -> Assert6/1
  be/1 -> Assert5/1
  r/1 -> Assert4/1
  w/1 -> Assert3/1
  a/1 -> Assert2/1
  d/1 -> Assert1/1
  Assert1/1 -> Configurable Subsystem/1(d)
  Assert2/1 -> Configurable Subsystem/2(a)
  Assert3/1 -> Configurable Subsystem/3(w)
  Assert4/1 -> Configurable Subsystem/4(r)
  Assert5/1 -> Configurable Subsystem/5(be)
  Assert6/1 -> Configurable Subsystem/6(adlocb_in)
  Assert7/1 -> q/1
  Assert8/1 -> qv/1
  Assert9/1 -> adlocb_out/1

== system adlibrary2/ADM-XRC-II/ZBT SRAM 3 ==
  d : Inport
  a : Inport  Port=2
  w : Inport  Port=3
  r : Inport  Port=4
  be : Inport  Port=5
  adlocb_in : Inport  Port=6
  Assert{1..9} (9 alike) : xbsIndex_r4/Assert  assert_type=off  type_source=Explicitly  arith_type="Signed  (2's comp)"  n_bits=16  bin_pt=14  assert_rate=on  rate_source=Explicitly  period=1  output_port=on  block_type=assert
  Configurable Subsystem : Subsystem  Tag=configX  BlockChoice=ZBT SRAM 32Bit Simulation
  q : Outport
  qv : Outport  Port=2
  adlocb_out : Outport  Port=3
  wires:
  Configurable Subsystem/3(adlocb_out) -> Assert9/1
  Configurable Subsystem/2(qv) -> Assert8/1
  Configurable Subsystem/1(q) -> Assert7/1
  adlocb_in/1 -> Assert6/1
  be/1 -> Assert5/1
  r/1 -> Assert4/1
  w/1 -> Assert3/1
  a/1 -> Assert2/1
  d/1 -> Assert1/1
  Assert1/1 -> Configurable Subsystem/1(d)
  Assert2/1 -> Configurable Subsystem/2(a)
  Assert3/1 -> Configurable Subsystem/3(w)
  Assert4/1 -> Configurable Subsystem/4(r)
  Assert5/1 -> Configurable Subsystem/5(be)
  Assert6/1 -> Configurable Subsystem/6(adlocb_in)
  Assert7/1 -> q/1
  Assert8/1 -> qv/1
  Assert9/1 -> adlocb_out/1

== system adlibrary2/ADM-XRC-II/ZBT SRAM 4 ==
  d : Inport
  a : Inport  Port=2
  w : Inport  Port=3
  r : Inport  Port=4
  be : Inport  Port=5
  adlocb_in : Inport  Port=6
  Assert{1..9} (9 alike) : xbsIndex_r4/Assert  assert_type=off  type_source=Explicitly  arith_type="Signed  (2's comp)"  n_bits=16  bin_pt=14  assert_rate=on  rate_source=Explicitly  period=1  output_port=on  block_type=assert
  Configurable Subsystem : Subsystem  Tag=configX  BlockChoice=ZBT SRAM 32Bit Simulation
  q : Outport
  qv : Outport  Port=2
  adlocb_out : Outport  Port=3
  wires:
  Configurable Subsystem/3(adlocb_out) -> Assert9/1
  Configurable Subsystem/2(qv) -> Assert8/1
  Configurable Subsystem/1(q) -> Assert7/1
  adlocb_in/1 -> Assert6/1
  be/1 -> Assert5/1
  r/1 -> Assert4/1
  w/1 -> Assert3/1
  a/1 -> Assert2/1
  d/1 -> Assert1/1
  Assert1/1 -> Configurable Subsystem/1(d)
  Assert2/1 -> Configurable Subsystem/2(a)
  Assert3/1 -> Configurable Subsystem/3(w)
  Assert4/1 -> Configurable Subsystem/4(r)
  Assert5/1 -> Configurable Subsystem/5(be)
  Assert6/1 -> Configurable Subsystem/6(adlocb_in)
  Assert7/1 -> q/1
  Assert8/1 -> qv/1
  Assert9/1 -> adlocb_out/1

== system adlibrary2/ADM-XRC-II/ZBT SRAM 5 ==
  d : Inport
  a : Inport  Port=2
  w : Inport  Port=3
  r : Inport  Port=4
  be : Inport  Port=5
  adlocb_in : Inport  Port=6
  Assert{1..9} (9 alike) : xbsIndex_r4/Assert  assert_type=off  type_source=Explicitly  arith_type="Signed  (2's comp)"  n_bits=16  bin_pt=14  assert_rate=on  rate_source=Explicitly  period=1  output_port=on  block_type=assert
  Configurable Subsystem : Subsystem  Tag=configX  BlockChoice=ZBT SRAM 32Bit Simulation
  q : Outport
  qv : Outport  Port=2
  adlocb_out : Outport  Port=3
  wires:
  Configurable Subsystem/3(adlocb_out) -> Assert9/1
  Configurable Subsystem/2(qv) -> Assert8/1
  Configurable Subsystem/1(q) -> Assert7/1
  adlocb_in/1 -> Assert6/1
  be/1 -> Assert5/1
  r/1 -> Assert4/1
  w/1 -> Assert3/1
  a/1 -> Assert2/1
  d/1 -> Assert1/1
  Assert1/1 -> Configurable Subsystem/1(d)
  Assert2/1 -> Configurable Subsystem/2(a)
  Assert3/1 -> Configurable Subsystem/3(w)
  Assert4/1 -> Configurable Subsystem/4(r)
  Assert5/1 -> Configurable Subsystem/5(be)
  Assert6/1 -> Configurable Subsystem/6(adlocb_in)
  Assert7/1 -> q/1
  Assert8/1 -> qv/1
  Assert9/1 -> adlocb_out/1

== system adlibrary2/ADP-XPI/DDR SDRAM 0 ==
  cache_data_in : Inport
  cache_addr : Inport  Port=2
  cache_write : Inport  Port=3
  ddr_page : Inport  Port=4
  ddr_addr : Inport  Port=5
  ddr_read : Inport  Port=6
  ddr_write : Inport  Port=7
  Assert{1..7,9..10} (9 alike) : xbsIndex_r4/Assert  assert_type=off  type_source=Explicitly  arith_type="Signed  (2's comp)"  n_bits=16  bin_pt=14  assert_rate=on  rate_source=Explicitly  period=1  output_port=on  block_type=assert
  Configurable Subsystem : Subsystem  Tag=configX  BlockChoice=DDR SDRAM 64bit Simulation  mask{memsize=memsize}
      mask prompts: memsize "Simulation Ram Size (Mb)"
  cache_data_out : Outport
  ddr_busy : Outport  Port=2
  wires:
  Assert10/1 -> ddr_busy/1
  Assert9/1 -> cache_data_out/1
  Assert6/1 -> Configurable Subsystem/6(ddr_read)
  Assert5/1 -> Configurable Subsystem/5(ddr_addr)
  Assert4/1 -> Configurable Subsystem/4(ddr_page)
  Assert3/1 -> Configurable Subsystem/3(cache_write)
  Assert2/1 -> Configurable Subsystem/2(cache_addr)
  Assert1/1 -> Configurable Subsystem/1(cache_data_in)
  ddr_write/1 -> Assert7/1
  ddr_read/1 -> Assert6/1
  ddr_addr/1 -> Assert5/1
  ddr_page/1 -> Assert4/1
  cache_write/1 -> Assert3/1
  cache_addr/1 -> Assert2/1
  cache_data_in/1 -> Assert1/1
  Configurable Subsystem/1(cache_data_out) -> Assert9/1
  Configurable Subsystem/2(ddr_busy) -> Assert10/1
  Assert7/1 -> Configurable Subsystem/7(ddr_write)

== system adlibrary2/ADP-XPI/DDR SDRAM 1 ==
  cache_data_in : Inport
  cache_addr : Inport  Port=2
  cache_write : Inport  Port=3
  ddr_page : Inport  Port=4
  ddr_addr : Inport  Port=5
  ddr_read : Inport  Port=6
  ddr_write : Inport  Port=7
  Assert{1..7,9..10} (9 alike) : xbsIndex_r4/Assert  assert_type=off  type_source=Explicitly  arith_type="Signed  (2's comp)"  n_bits=16  bin_pt=14  assert_rate=on  rate_source=Explicitly  period=1  output_port=on  block_type=assert
  Configurable Subsystem : Subsystem  Tag=configX  BlockChoice=DDR SDRAM 64bit Simulation  mask{memsize=memsize}
      mask prompts: memsize "Simulation Ram Size (Mb)"
  cache_data_out : Outport
  ddr_busy : Outport  Port=2
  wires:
  Assert7/1 -> Configurable Subsystem/7(ddr_write)
  Configurable Subsystem/2(ddr_busy) -> Assert10/1
  Configurable Subsystem/1(cache_data_out) -> Assert9/1
  cache_data_in/1 -> Assert1/1
  cache_addr/1 -> Assert2/1
  cache_write/1 -> Assert3/1
  ddr_page/1 -> Assert4/1
  ddr_addr/1 -> Assert5/1
  ddr_read/1 -> Assert6/1
  ddr_write/1 -> Assert7/1
  Assert1/1 -> Configurable Subsystem/1(cache_data_in)
  Assert2/1 -> Configurable Subsystem/2(cache_addr)
  Assert3/1 -> Configurable Subsystem/3(cache_write)
  Assert4/1 -> Configurable Subsystem/4(ddr_page)
  Assert5/1 -> Configurable Subsystem/5(ddr_addr)
  Assert6/1 -> Configurable Subsystem/6(ddr_read)
  Assert9/1 -> cache_data_out/1
  Assert10/1 -> ddr_busy/1

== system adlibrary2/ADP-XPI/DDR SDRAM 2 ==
  cache_data_in : Inport
  cache_addr : Inport  Port=2
  cache_write : Inport  Port=3
  ddr_page : Inport  Port=4
  ddr_addr : Inport  Port=5
  ddr_read : Inport  Port=6
  ddr_write : Inport  Port=7
  Assert{1..7,9..10} (9 alike) : xbsIndex_r4/Assert  assert_type=off  type_source=Explicitly  arith_type="Signed  (2's comp)"  n_bits=16  bin_pt=14  assert_rate=on  rate_source=Explicitly  period=1  output_port=on  block_type=assert
  Configurable Subsystem : Subsystem  Tag=configX  BlockChoice=DDR SDRAM 64bit Simulation  mask{memsize=memsize}
      mask prompts: memsize "Simulation Ram Size (Mb)"
  cache_data_out : Outport
  ddr_busy : Outport  Port=2
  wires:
  Assert10/1 -> ddr_busy/1
  Assert9/1 -> cache_data_out/1
  Assert6/1 -> Configurable Subsystem/6(ddr_read)
  Assert5/1 -> Configurable Subsystem/5(ddr_addr)
  Assert4/1 -> Configurable Subsystem/4(ddr_page)
  Assert3/1 -> Configurable Subsystem/3(cache_write)
  Assert2/1 -> Configurable Subsystem/2(cache_addr)
  Assert1/1 -> Configurable Subsystem/1(cache_data_in)
  ddr_write/1 -> Assert7/1
  ddr_read/1 -> Assert6/1
  ddr_addr/1 -> Assert5/1
  ddr_page/1 -> Assert4/1
  cache_write/1 -> Assert3/1
  cache_addr/1 -> Assert2/1
  cache_data_in/1 -> Assert1/1
  Configurable Subsystem/1(cache_data_out) -> Assert9/1
  Configurable Subsystem/2(ddr_busy) -> Assert10/1
  Assert7/1 -> Configurable Subsystem/7(ddr_write)

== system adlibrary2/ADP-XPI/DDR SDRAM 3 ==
  cache_data_in : Inport
  cache_addr : Inport  Port=2
  cache_write : Inport  Port=3
  ddr_page : Inport  Port=4
  ddr_addr : Inport  Port=5
  ddr_read : Inport  Port=6
  ddr_write : Inport  Port=7
  Assert{1..7,9..10} (9 alike) : xbsIndex_r4/Assert  assert_type=off  type_source=Explicitly  arith_type="Signed  (2's comp)"  n_bits=16  bin_pt=14  assert_rate=on  rate_source=Explicitly  period=1  output_port=on  block_type=assert
  Configurable Subsystem : Subsystem  Tag=configX  BlockChoice=DDR SDRAM 64bit Simulation  mask{memsize=memsize}
      mask prompts: memsize "Simulation Ram Size (Mb)"
  cache_data_out : Outport
  ddr_busy : Outport  Port=2
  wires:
  Assert7/1 -> Configurable Subsystem/7(ddr_write)
  Configurable Subsystem/2(ddr_busy) -> Assert10/1
  Configurable Subsystem/1(cache_data_out) -> Assert9/1
  cache_data_in/1 -> Assert1/1
  cache_addr/1 -> Assert2/1
  cache_write/1 -> Assert3/1
  ddr_page/1 -> Assert4/1
  ddr_addr/1 -> Assert5/1
  ddr_read/1 -> Assert6/1
  ddr_write/1 -> Assert7/1
  Assert1/1 -> Configurable Subsystem/1(cache_data_in)
  Assert2/1 -> Configurable Subsystem/2(cache_addr)
  Assert3/1 -> Configurable Subsystem/3(cache_write)
  Assert4/1 -> Configurable Subsystem/4(ddr_page)
  Assert5/1 -> Configurable Subsystem/5(ddr_addr)
  Assert6/1 -> Configurable Subsystem/6(ddr_read)
  Assert9/1 -> cache_data_out/1
  Assert10/1 -> ddr_busy/1

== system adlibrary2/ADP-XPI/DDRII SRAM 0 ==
  d : Inport
  a : Inport  Port=2
  w : Inport  Port=3
  r : Inport  Port=4
  be : Inport  Port=5
  adlocb_in : Inport  Port=6
  Assert{1..9} (9 alike) : xbsIndex_r4/Assert  assert_type=off  type_source=Explicitly  arith_type="Signed  (2's comp)"  n_bits=16  bin_pt=14  assert_rate=on  rate_source=Explicitly  period=1  output_port=on  block_type=assert
  Configurable Subsystem : Subsystem  Tag=configX  BlockChoice=DDRII SRAM Simulation
  q : Outport
  qv : Outport  Port=2
  adlocb_out : Outport  Port=3
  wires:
  Assert9/1 -> adlocb_out/1
  Assert8/1 -> qv/1
  Assert7/1 -> q/1
  Assert6/1 -> Configurable Subsystem/6(adlocb_in)
  Assert5/1 -> Configurable Subsystem/5(be)
  Assert4/1 -> Configurable Subsystem/4(r)
  Assert3/1 -> Configurable Subsystem/3(w)
  Assert2/1 -> Configurable Subsystem/2(a)
  Assert1/1 -> Configurable Subsystem/1(d)
  Configurable Subsystem/2(qv) -> Assert8/1
  Configurable Subsystem/3(adlocb_out) -> Assert9/1
  adlocb_in/1 -> Assert6/1
  be/1 -> Assert5/1
  r/1 -> Assert4/1
  w/1 -> Assert3/1
  a/1 -> Assert2/1
  d/1 -> Assert1/1
  Configurable Subsystem/1(q) -> Assert7/1

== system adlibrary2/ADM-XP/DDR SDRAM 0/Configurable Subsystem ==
  cache_data_in : Inport
  cache_addr : Inport  Port=2
  cache_write : Inport  Port=3
  ddr_page : Inport  Port=4
  ddr_addr : Inport  Port=5
  ddr_read : Inport  Port=6
  ddr_write : Inport  Port=7
  adlocb_in : Inport  Port=8
  DDR SDRAM 32bit Simulation : adlibrary2_ddr_xpl/DDR SDRAM 32bit Simulation  memsize=memsize
  cache_data_out : Outport
  ddr_busy : Outport  Port=2
  adlocb_out : Outport  Port=3
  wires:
  cache_data_in/1 -> DDR SDRAM 32bit Simulation/1
  cache_addr/1 -> DDR SDRAM 32bit Simulation/2
  cache_write/1 -> DDR SDRAM 32bit Simulation/3
  ddr_page/1 -> DDR SDRAM 32bit Simulation/4
  ddr_addr/1 -> DDR SDRAM 32bit Simulation/5
  ddr_read/1 -> DDR SDRAM 32bit Simulation/6
  ddr_write/1 -> DDR SDRAM 32bit Simulation/7
  adlocb_in/1 -> DDR SDRAM 32bit Simulation/8
  DDR SDRAM 32bit Simulation/1 -> cache_data_out/1
  DDR SDRAM 32bit Simulation/2 -> ddr_busy/1
  DDR SDRAM 32bit Simulation/3 -> adlocb_out/1

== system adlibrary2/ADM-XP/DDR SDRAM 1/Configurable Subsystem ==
  cache_data_in : Inport
  cache_addr : Inport  Port=2
  cache_write : Inport  Port=3
  ddr_page : Inport  Port=4
  ddr_addr : Inport  Port=5
  ddr_read : Inport  Port=6
  ddr_write : Inport  Port=7
  adlocb_in : Inport  Port=8
  DDR SDRAM 32bit Simulation : adlibrary2_ddr_xpl/DDR SDRAM 32bit Simulation  memsize=memsize
  cache_data_out : Outport
  ddr_busy : Outport  Port=2
  adlocb_out : Outport  Port=3
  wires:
  cache_data_in/1 -> DDR SDRAM 32bit Simulation/1
  cache_addr/1 -> DDR SDRAM 32bit Simulation/2
  cache_write/1 -> DDR SDRAM 32bit Simulation/3
  ddr_page/1 -> DDR SDRAM 32bit Simulation/4
  ddr_addr/1 -> DDR SDRAM 32bit Simulation/5
  ddr_read/1 -> DDR SDRAM 32bit Simulation/6
  ddr_write/1 -> DDR SDRAM 32bit Simulation/7
  adlocb_in/1 -> DDR SDRAM 32bit Simulation/8
  DDR SDRAM 32bit Simulation/1 -> cache_data_out/1
  DDR SDRAM 32bit Simulation/2 -> ddr_busy/1
  DDR SDRAM 32bit Simulation/3 -> adlocb_out/1

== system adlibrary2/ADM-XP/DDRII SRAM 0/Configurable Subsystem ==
  d : Inport
  a : Inport  Port=2
  w : Inport  Port=3
  r : Inport  Port=4
  be : Inport  Port=5
  adlocb_in : Inport  Port=6
  DDRII SRAM Simulation : adlibrary2_d2sram_0/DDRII SRAM Simulation
  q : Outport
  qv : Outport  Port=2
  adlocb_out : Outport  Port=3
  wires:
  d/1 -> DDRII SRAM Simulation/1
  a/1 -> DDRII SRAM Simulation/2
  w/1 -> DDRII SRAM Simulation/3
  r/1 -> DDRII SRAM Simulation/4
  be/1 -> DDRII SRAM Simulation/5
  adlocb_in/1 -> DDRII SRAM Simulation/6
  DDRII SRAM Simulation/1 -> q/1
  DDRII SRAM Simulation/2 -> qv/1
  DDRII SRAM Simulation/3 -> adlocb_out/1

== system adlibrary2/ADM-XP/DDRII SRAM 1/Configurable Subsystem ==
  d : Inport
  a : Inport  Port=2
  w : Inport  Port=3
  r : Inport  Port=4
  be : Inport  Port=5
  adlocb_in : Inport  Port=6
  DDRII SRAM Simulation : adlibrary2_d2sram_0/DDRII SRAM Simulation
  q : Outport
  qv : Outport  Port=2
  adlocb_out : Outport  Port=3
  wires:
  d/1 -> DDRII SRAM Simulation/1
  a/1 -> DDRII SRAM Simulation/2
  w/1 -> DDRII SRAM Simulation/3
  r/1 -> DDRII SRAM Simulation/4
  be/1 -> DDRII SRAM Simulation/5
  adlocb_in/1 -> DDRII SRAM Simulation/6
  DDRII SRAM Simulation/1 -> q/1
  DDRII SRAM Simulation/2 -> qv/1
  DDRII SRAM Simulation/3 -> adlocb_out/1

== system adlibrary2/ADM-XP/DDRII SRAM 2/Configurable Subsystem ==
  d : Inport
  a : Inport  Port=2
  w : Inport  Port=3
  r : Inport  Port=4
  be : Inport  Port=5
  adlocb_in : Inport  Port=6
  DDRII SRAM Simulation : adlibrary2_d2sram_0/DDRII SRAM Simulation
  q : Outport
  qv : Outport  Port=2
  adlocb_out : Outport  Port=3
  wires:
  d/1 -> DDRII SRAM Simulation/1
  a/1 -> DDRII SRAM Simulation/2
  w/1 -> DDRII SRAM Simulation/3
  r/1 -> DDRII SRAM Simulation/4
  be/1 -> DDRII SRAM Simulation/5
  adlocb_in/1 -> DDRII SRAM Simulation/6
  DDRII SRAM Simulation/1 -> q/1
  DDRII SRAM Simulation/2 -> qv/1
  DDRII SRAM Simulation/3 -> adlocb_out/1

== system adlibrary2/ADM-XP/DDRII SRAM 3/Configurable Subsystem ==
  d : Inport
  a : Inport  Port=2
  w : Inport  Port=3
  r : Inport  Port=4
  be : Inport  Port=5
  adlocb_in : Inport  Port=6
  DDRII SRAM Simulation : adlibrary2_d2sram_0/DDRII SRAM Simulation
  q : Outport
  qv : Outport  Port=2
  adlocb_out : Outport  Port=3
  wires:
  d/1 -> DDRII SRAM Simulation/1
  a/1 -> DDRII SRAM Simulation/2
  w/1 -> DDRII SRAM Simulation/3
  r/1 -> DDRII SRAM Simulation/4
  be/1 -> DDRII SRAM Simulation/5
  adlocb_in/1 -> DDRII SRAM Simulation/6
  DDRII SRAM Simulation/1 -> q/1
  DDRII SRAM Simulation/2 -> qv/1
  DDRII SRAM Simulation/3 -> adlocb_out/1
